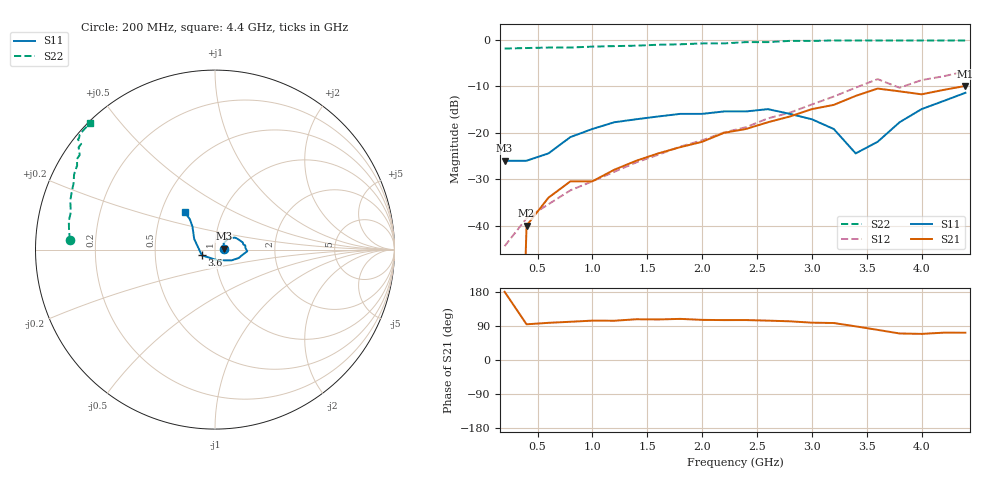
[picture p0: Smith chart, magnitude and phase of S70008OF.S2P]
!  MGS-70008 S PARAMETERS
!  "off" port  LAST UPDATED 07-22-92
# ghz s ma r 50
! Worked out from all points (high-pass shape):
!   22 points, 200 MHz to 4.4 GHz, reference 50 ohm
!   highest |S21| = -9.90 dB at 4.4 GHz (marker M1); lowest = -40.0 dB at 400 MHz (marker M2)
!   |S21| within 3 dB of the highest: 3.312 GHz to end of sweep
!   lowest |S11| = -26.0 dB at 200 MHz (marker M3), VSWR 1.11, Z = 55.2 + j0.54 ohm
!   |S11| at or under -10 dB: start of sweep to end of sweep
!   |S22| runs from -1.8 to -0.1 dB; largest |S21 - S12| = 0.16
!   S11 on the Smith chart (normalised r, x): 200 MHz: 1.10, +0.01; 3.6 GHz: 0.86, -0.05; 4.4 GHz: 0.66, +0.30
0.2  0.05 5.6  0 92.1  0.006 92.4  0.81 176.3
0.4  0.05 20.6  0.01 94.2  0.012 95.2  0.82 172.6
0.6  0.06 36.0  0.02 98.1  0.017 100.3  0.83 168.9
0.8  0.09 39.3  0.03 100.9  0.024 104.4  0.83 165.3
1  0.11 35.8  0.03 103.9  0.03 108.5  0.85 161.6
1.2  0.13 30.9  0.04 103.6  0.038 110.4  0.86 158.3
1.4  0.14 25.0  0.05 107.5  0.048 116.2  0.87 154.9
1.6  0.15 18.9  0.06 107.0  0.058 116.8  0.89 151.9
1.8  0.16 14.5  0.07 108.5  0.071 119.6  0.9 148.6
2  0.16 10.6  0.08 105.9  0.083 118.0  0.92 146.7
2.2  0.17 7.8  0.1 105.3  0.101 118.6  0.92 145.0
2.4  0.17 3.0  0.11 105.4  0.115 119.8  0.95 143.1
2.6  0.18 -2.9  0.13 103.9  0.143 120.4  0.95 141.7
2.8  0.16 -9.2  0.15 102.1  0.165 119.3  0.98 141.2
3  0.14 -19.6  0.18 98.5  0.202 116.4  0.98 140.6
3.2  0.11 -33.2  0.2 97.6  0.246 115.5  0.99 139.6
3.4  0.06 -78.5  0.25 88.8  0.307 105.1  0.99 139.0
3.6  0.08 -156.7  0.3 79.5  0.379 89.9  0.99 137.4
3.8  0.13 153.0  0.28 70.0  0.306 77.4  0.99 136.5
4  0.18 134.3  0.26 68.9  0.37 88.3  0.99 135.8
4.2  0.22 129.6  0.29 72.1  0.407 85.3  0.99 135.2
4.4  0.27 128.9  0.32 72.0  0.458 83.0  0.99 134.6
